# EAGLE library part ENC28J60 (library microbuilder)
ENC28J60 SPI Ethernet Controller Digikey: SSOP - ENC28J60/SS-ND
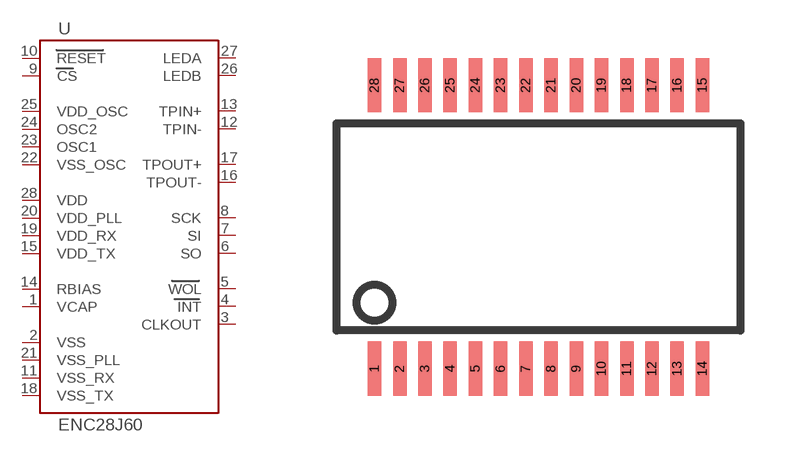
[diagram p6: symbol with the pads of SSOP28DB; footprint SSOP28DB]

Designator prefix U

## ENC28J60  [SSOP28DB]
1  VCAP
2  VSS
3  CLKOUT
4  INT
5  WOL
6  SO
7  SI
8  SCK
9  CS
10  RESET
11  VSS_RX
12  TPIN-
13  TPIN+
14  RBIAS
15  VDD_TX
16  TPOUT-
17  TPOUT+
18  VSS_TX
19  VDD_RX
20  VDD_PLL
21  VSS_PLL
22  VSS_OSC
23  OSC1
24  OSC2
25  VDD_OSC
26  LEDB
27  LEDA
28  VDD

## Footprint SSOP28DB (pad centres in mm)
Small Shrink Outline Package
smd 0.348 x 1.397: 1 -4.225,-3.656; 2 -3.575,-3.656; 3 -2.925,-3.656; 4 -2.275,-3.656; 5 -1.625,-3.656; 6 -0.975,-3.656; 7 -0.325,-3.656; 8 0.325,-3.656; 9 0.975,-3.656; 10 1.625,-3.656; 11 2.275,-3.656; 12 2.925,-3.656; 13 3.575,-3.656; 14 4.225,-3.656; 15 4.225,3.656; 16 3.575,3.656; 17 2.925,3.656; 18 2.275,3.656; 19 1.625,3.656; 20 0.975,3.656; 21 0.325,3.656; 22 -0.325,3.656; 23 -0.975,3.656; 24 -1.625,3.656; 25 -2.275,3.656; 26 -2.925,3.656; 27 -3.575,3.656; 28 -4.225,3.656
